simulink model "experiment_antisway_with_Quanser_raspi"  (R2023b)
settings: configuration reference "FRE_experiment_config_PIL" (kept in a data dictionary, not in this file)
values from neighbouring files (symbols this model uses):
  FRE_time_step = 0.005
                
                    
                        1
                        Auto
                        
                        
                        -1.0
                        0
                        Simulink
                        Parameter
                        Default    [run_FRE_data.sldd]
libraries: simulink x2, SignalEditorBlockLib x1

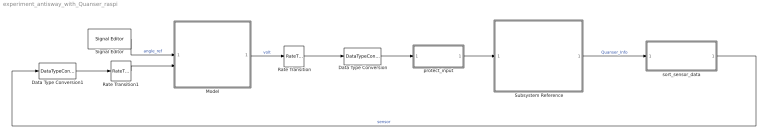
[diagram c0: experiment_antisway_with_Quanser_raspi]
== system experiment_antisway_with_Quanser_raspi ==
  Data Type Conversion : DataTypeConversion  OutDataTypeStr=double
  Data Type Conversion1 : DataTypeConversion  OutDataTypeStr=single
  Model : ModelReference  ModelNameDialog=control_pendulum_angle.slx  SimulationMode=Normal  ModelReferenceVersion=1.70
  Rate Transition : RateTransition
  Rate Transition1 : RateTransition  OutPortSampleTime=FRE_time_step
  Signal Editor : SignalEditorBlockLib/Signal Editor  FileName=pendulum_reference_data.mat  ActiveScenario=Step_sequence  ActiveSignal=angle_ref  IsBus=off  OutputBusObjectStr=Bus: BusObject  SampleTime=FRE_time_step  Interpolate=off  ZeroCross=off  OutputAfterFinalValue=Holding final value  Unit=inherit  PreserveSignalName=on  ApplySigPropsToAllScenarios=on  ApplySigPropsToAllSignals=on
  Subsystem Reference : Subsystem  ReferencedSubsystem=raspi_Quanser
  protect_input : Subsystem  ReferencedSubsystem=protect_input
  sort_sensor_data : Subsystem
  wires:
  Rate Transition/1 -> Data Type Conversion/1
  Rate Transition1/1 -> Model/2
  Data Type Conversion1/1 -> Rate Transition1/1
  Model/1 -> Rate Transition/1  "volt"
  Data Type Conversion/1 -> protect_input/1
  sort_sensor_data/1(sensor) -> Data Type Conversion1/1  "sensor"
  Subsystem Reference/1 -> sort_sensor_data/1(Quanser_Info)  "Quanser_Info"
  protect_input/1 -> Subsystem Reference/1
  Signal Editor/1 -> Model/1  "angle_ref"

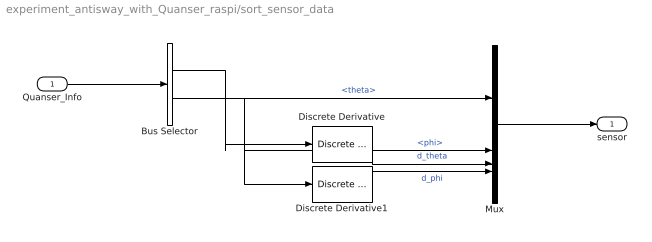
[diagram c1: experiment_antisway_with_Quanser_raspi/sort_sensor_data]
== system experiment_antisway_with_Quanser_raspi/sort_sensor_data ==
  Quanser_Info : Inport
  Bus Selector : BusSelector  OutputSignals=theta,phi
  Discrete Derivative : simulink/Discrete/Discrete Derivative  gainval=1.0  ICPrevScaledInput=0.0  OutMin=[]  OutMax=[]  OutDataType=fixdt(1, 16)  OutScaling=2^-10  DoSatur=off
  Discrete Derivative1 : simulink/Discrete/Discrete Derivative  gainval=1.0  ICPrevScaledInput=0.0  OutMin=[]  OutMax=[]  OutDataType=fixdt(1, 16)  OutScaling=2^-10  DoSatur=off
  Mux : Mux
  sensor : Outport
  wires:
  Quanser_Info/1 -> Bus Selector/1
  Bus Selector/1 -> Discrete Derivative/1, Mux/1  "<theta>"
  Bus Selector/2 -> Discrete Derivative1/1, Mux/2  "<phi>"
  Discrete Derivative1/1 -> Mux/4  "d_phi"
  Mux/1 -> sensor/1
  Discrete Derivative/1 -> Mux/3  "d_theta"
